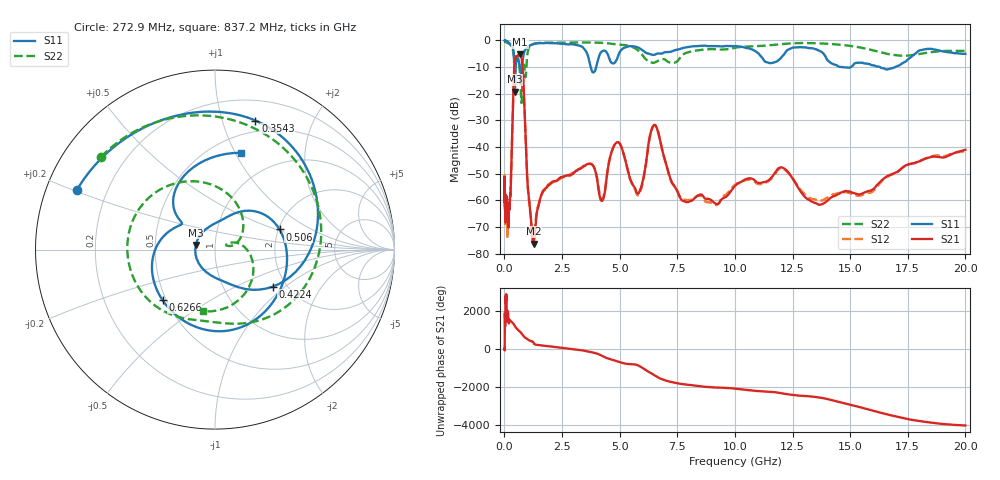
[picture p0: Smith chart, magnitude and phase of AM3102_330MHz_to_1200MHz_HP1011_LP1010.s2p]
! Date/Time: Tue, Sep 11, 2018 5:20 PM
! Network Analyzer: Agilent Technologies E8362B Rev: A.07.50.63
! Sweep from 0.010 to 20.000 GHz, 1601 Points, Sweep Type: LOG
! Power Supply: 4.949 V, 0.001 A
# Hz S DB R 50
!freq MagS11 AngS11 MagS21 AngS21 MagS12 AngS12 MagS22 AngS22
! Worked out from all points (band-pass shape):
!   1601 points, 10 MHz to 20 GHz, reference 50 ohm
!   highest |S21| = -5.19 dB at 676.1 MHz (marker M1); lowest = -76.2 dB at 1.272 GHz (marker M2)
!   |S21| within 3 dB of the highest: 442.1 MHz to 771.8 MHz (329.7 MHz wide, 54.3 % of centre)
!   lowest |S11| = -19.2 dB at 455.8 MHz (marker M3), VSWR 1.25, Z = 40.3 + j2.06 ohm
!   |S11| at or under -10 dB: 3.745 GHz to 3.983 GHz (237.8 MHz wide, 6.15 % of centre); 14.64 GHz to 15.03 GHz (386.7 MHz wide, 2.61 % of centre); 16.29 GHz to 16.95 GHz (663.4 MHz wide, 3.99 % of centre)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
!   |S22| runs from -23.5 to -0.2 dB; largest |S21 - S12| = 0.0099
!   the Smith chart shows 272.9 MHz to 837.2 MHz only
!   S11 on the Smith chart (normalised r, x): 272.9 MHz: 0.09, +0.20; 354.3 MHz: 0.39, +1.29; 422.4 MHz: 1.70, -0.82; 506 MHz: 2.03, +0.53; 626.6 MHz: 0.48, -0.32; 837.2 MHz: 0.67, +1.06
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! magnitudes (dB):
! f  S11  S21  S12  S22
! 10 MHz  0.0  -51.4  -51.4  -0.2
! 35.55 MHz  0.0  -63.1  -64.5  -0.4
! 126.4 MHz  -0.4  -66.7  -73.2  -0.9
! 272.9 MHz  -1.5  -55.8  -55.5  -1.7
! 354.3 MHz  -2.5  -30.4  -30.6  -3.2
! 422.4 MHz  -8.4  -11.2  -11.3  -6.3
! 447.2 MHz  -18.5  -7.7  -7.7  -7.8
! 455.8 MHz  -19.2  -7.1  -7.1  -7.9
! 506 MHz  -8.5  -6.0  -6.1  -6.6
! 626.6 MHz  -7.8  -5.3  -5.4  -8.2
! 676.1 MHz  -10.0  -5.2  -5.2  -12.2
! 837.2 MHz  -5.1  -17.8  -17.9  -9.1
! 1.272 GHz  -1.4  -76.2  -75.5  -1.3
! 1.59 GHz  -1.0  -58.3  -58.3  -0.9
! 3.668 GHz  -7.2  -46.3  -46.2  -0.8
! 4.23 GHz  -4.1  -60.2  -59.6  -0.9
! 4.902 GHz  -6.6  -38.2  -38.2  -1.5
! 5.652 GHz  -2.3  -55.2  -55.5  -2.9
! 6.518 GHz  -5.4  -31.6  -31.8  -8.3
! 7.92 GHz  -2.5  -60.6  -59.9  -4.6
! 13.81 GHz  -4.6  -61.3  -60.0  -1.2
! 20 GHz  -5.0  -41.0  -41.6  -3.9
